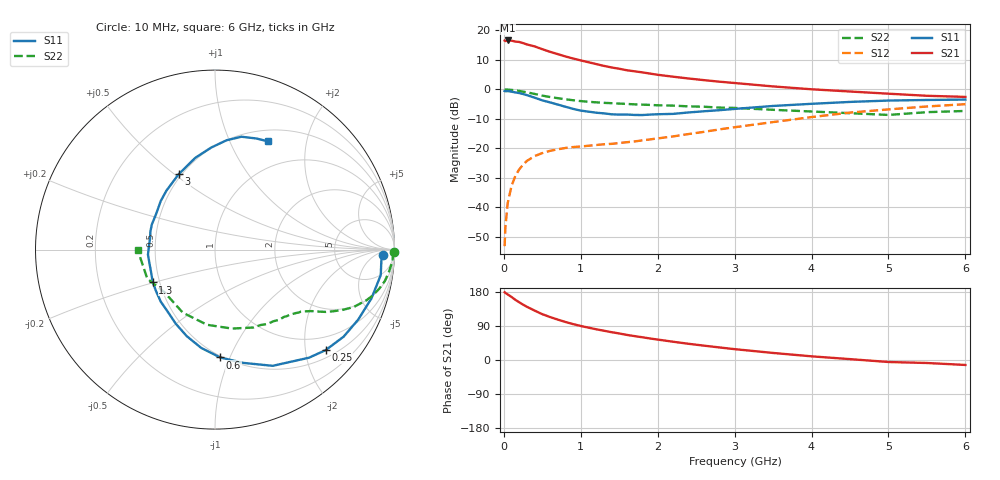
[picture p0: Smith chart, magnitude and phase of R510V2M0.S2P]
! SIEMENS Small Signal Semiconductors
! BFR183
! Si NPN RF Bipolar Junction Transistor in SOT23
! VCE = 10 V  IC = 2 mA
! Common Emitter S-Parameters:  May  1996
# GHz  S  MA  R  50
!  f  S11  S21  S12  S22
! GHz  MAG  ANG  MAG  ANG  MAG  ANG  MAG  ANG
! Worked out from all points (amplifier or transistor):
!   36 points, 10 MHz to 6 GHz, reference 50 ohm
!   highest |S21| = 16.6 dB at 50 MHz (marker M1)
!   |S21| within 3 dB of that: start of sweep to 504.8 MHz
!   unconditionally stable (mu >= 1): 1.423 GHz to 2.896 GHz
!   at 250 MHz: K = 0.22, MSG = 20.6 dB, |S12| = -25.5 dB
!   at 1.4 GHz: K = 0.99, MSG = 12.9 dB, |S12| = -18.5 dB
!   at 6 GHz: K = 0.89, MSG = 1.2 dB, |S12| = -5.0 dB
!   S11 on the Smith chart (normalised r, x): 10 MHz: 26, -12; 250 MHz: 0.67, -2.43; 600 MHz: 0.49, -0.92; 1.3 GHz: 0.46, -0.20; 3 GHz: 0.48, +0.52; 6 GHz: 0.64, +1.40
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0.01  0.9378 -1.7  6.698 178.8  0.0022 90.1  0.9948 -0.7
0.02  0.9288 -3.5  6.57 177.0  0.0046 84.0  0.9921 -1.4
0.05  0.9343 -8.7  6.739 173.0  0.0118 84.2  0.9911 -3.6
0.1  0.9132 -17.3  6.674 166.3  0.0231 79.7  0.9777 -7.1
0.15  0.8882 -26.0  6.452 158.7  0.0342 75.3  0.9629 -10.4
0.2  0.8654 -34.1  6.356 152.3  0.044 70.9  0.9405 -13.4
0.25  0.8332 -42.2  6.077 146.1  0.053 66.5  0.9142 -16.3
0.3  0.7981 -49.0  5.773 140.4  0.0613 63.5  0.8898 -18.5
0.4  0.7229 -63.6  5.341 130.4  0.074 56.9  0.8362 -22.5
0.5  0.6509 -75.9  4.794 120.9  0.0832 52.5  0.7831 -25.5
0.6  0.6013 -87.3  4.331 113.4  0.0908 49.1  0.7418 -27.6
0.8  0.5071 -108.1  3.608 100.4  0.1014 44.7  0.6793 -30.6
0.9  0.4672 -117.9  3.334 94.7  0.1053 44.1  0.6536 -31.7
1.1  0.419 -136.1  2.881 85.4  0.1107 43.6  0.6162 -33.9
1.3  0.3919 -152.2  2.501 77.3  0.1173 44.2  0.5907 -35.8
1.7  0.3682 176.2  2.022 63.0  0.131 47.9  0.5566 -40.3
2.2  0.3839 148.4  1.639 48.2  0.1593 52.2  0.5302 -47.4
3  0.4662 115.8  1.28 28.6  0.2278 53.8  0.4842 -63.7
3.5  0.5231 102.1  1.121 18.6  0.279 50.8  0.45 -77.9
4.5  0.6124 84.0  0.919 2.3  0.4039 40.1  0.3946 -117.0
5.5  0.6606 69.6  0.778 -7.9  0.5126 26.1  0.4106 -156.8
6  0.671 64.1  0.745 -13.1  0.5604 17.0  0.4305 -179.6
